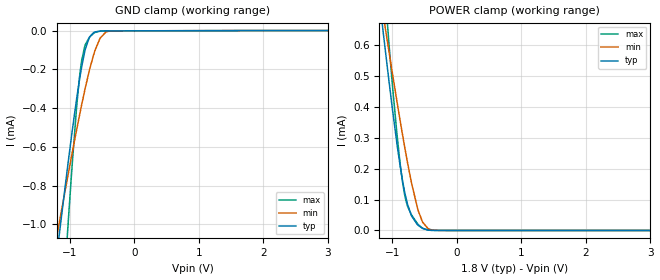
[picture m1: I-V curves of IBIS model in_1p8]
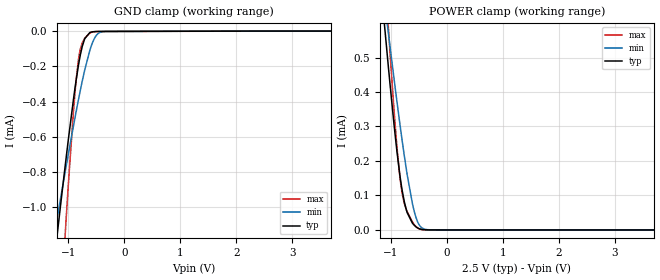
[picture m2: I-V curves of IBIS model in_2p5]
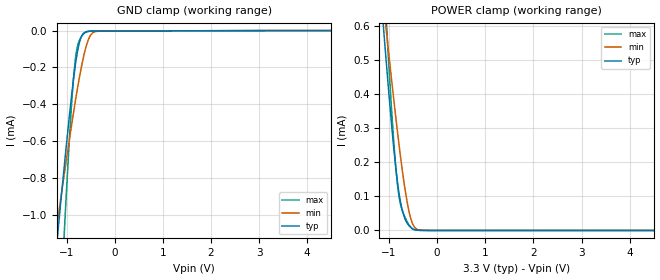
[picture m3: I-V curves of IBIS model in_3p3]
| Texas Instruments Incorporated
| High Speed, Robust EMC Reinforced Dual-Channel Digital Isolators
[IBIS Ver]   4.1
[File name]   iso6521.ibs
[File Rev]   1.0
[Date]   11/6/2023
[Source]
| Texas Instruments Incorporated.
| Analog-eLab Design Center, HPA
| 12500 TI Blvd
| Dallas, TX -75243
[Notes]   Revision History:
| Rev 1.0: 11/6/2023
| - Initial version of the model
|* EXCEPTION:   *
|* - For in_* and en_* models there will be leakage current in   *
|*   GROUND clamp because of a resistor(RH2) connected to pad.   *
|* - For inf_* models there will be leakage current in POWER clamp  *
|*   because of a resistor(R1) connected to pad.   *
[Disclaimer]
| This model is designed as an aid for customers of Texas Instruments.
| TI and its licensors and suppliers make no warranties, either expressed
| or implied, with respect to this  model, including the warranties of
| merchantability or fitness for a particular purpose. The model is
| provided solely on an "as is" basis. The entire risk as to its quality
| and performance is with the customer.
[Copyright]
(C) Copyright 2016 Texas Instruments Incorporated.All rights reserved.
| Marketing part#   Digital Voltage Range   Package-type   #pins
| IS07721DW   2.25V-5.5V   SOIC   16
| IS07721DWR   2.25V-5.5V   SOIC   16
|  Component ISO6521 8-Pin REU DFN package
|  Part # ISO6521
[Component]   IS06521DFN
[Manufacturer]   TI
[Package]   |8 REU - DFN package
|   typ   min   max
R_pkg   0.0519   0.0296   0.0664
L_pkg   1.5958n   1.4642n   1.7808n
C_pkg   0.3172p   0.2996p   0.3431p
[Pin]  signal_name   model_name   R_pin   L_pin   C_pin
1   VCC1   POWER   0.03706  1.83239n  0.42768p
2   OUTA   OUT   0.07937  1.93924n  0.37453p
3   INB   IN   0.08295  1.99423n  0.37759p
4   GND1   GND   0.06024  2.20170n  0.40515p
5   GND2   GND   0.06024  2.22600n  0.40576p
6   OUTB   OUT   0.08295  1.99420n  0.37782p
7   INA   IN   0.07937  1.93924n  0.37472p
8   VCC2   POWER   0.03703  1.83026n  0.42888p
|  Component ISO6521F 8-Pin REU DFN package
|  Part # ISO6521F
[Component]   IS06521FDFN
[Manufacturer]   TI
[Package]   |8 REU - DFN package
|   typ   min   max
R_pkg   0.0519   0.0296   0.0664
L_pkg   1.5958n   1.4642n   1.7808n
C_pkg   0.3172p   0.2996p   0.3431p
[Pin]  signal_name   model_name   R_pin   L_pin   C_pin
1   VCC1   POWER   0.03706  1.83239n  0.42768p
2   OUTA   OUT   0.07937  1.93924n  0.37453p
3   INB   INF   0.08295  1.99423n  0.37759p
4   GND1   GND   0.06024  2.20170n  0.40515p
5   GND2   GND   0.06024  2.22600n  0.40576p
6   OUTB   OUT   0.08295  1.99420n  0.37782p
7   INA   INF   0.07937  1.93924n  0.37472p
8   VCC2   POWER   0.03703  1.83026n  0.42888p
|   Model Selectors
[Model Selector] IN
in_1p8   1.8V digital Input
in_2p5   2.5V digital Input
in_3p3   3.3V digital Input
in_5   5.0V digital Input
[Model Selector] INF
inf_1p8   1.8V digital Input
inf_2p5   2.5V digital Input
inf_3p3   3.3V digital Input
inf_5   5.0V digital Input
[Model Selector] OUT
out_1p8   1.8V digital Output
out_2p5   2.5V digital Output
out_3p3   3.3V digital Output
out_5   5.0V digital Output
| Models and submodels in the file (12): in_1p8 (Input), in_2p5 (Input), in_3p3 (Input), in_5 (Input), inf_1p8 (Input), inf_2p5 (Input), inf_3p3 (Input), inf_5 (Input), out_1p8 (3-state), out_2p5 (3-state), out_3p3 (3-state), out_5 (3-state)
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|   in_2p5 Model
[Model]   in_1p8
Model_type   Input
Vinl = 0.54
Vinh = 1.26
|   typ   min   max
C_comp   0.00095pF   0.00076pF   0.0142pF
[Model spec]
|subparameter
Vinl   0.54   0.513   0.567
Vinh   1.26   1.197   1.323
| Where nom  PVT is Nominal Process, 2.5V, 27C
|   Fast PVT is Strong Process,  2.75V, -55C
|   Slow PVT is Weak Process,   2.25V, 150C
[Voltage Range]   1.8   1.71   1.89
|Ambient Temperature   25   125   -55
|Junction Temperature
[Temperature Range]   27   150   -40
[Power Clamp Reference]   1.8   1.71   1.89
[GND Clamp Reference]   0   0   0
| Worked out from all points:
|   GND clamp passes 1 mA (typ) near -1.14 V on its own axis
|   POWER clamp passes 1 mA (typ) near -1.34 V on its own axis
[GND Clamp]
|   Voltage   I(typ)   I(min)   I(max)
-1.8V     -2.874mA   -2.195mA   -5.336mA
-1.184V   -1.11mA    -1.03mA    -1.821mA
-1.163V   -1.051mA   -990.6uA   -1.705mA
-1.028V   -686uA     -745.6uA   -1.004mA
-898.2mV  -361.3uA   -518.9uA   -411.1uA
-828mV    -209.5uA   -402uA     -181.4uA
-757.8mV  -93.79uA   -292.1uA   -71.12uA
-698.4mV  -36.2uA    -207.5uA   -35.59uA
-633.6mV  -10.97uA   -127.9uA   -14.52uA
-531mV    -2.469uA   -39.62uA   -2.975uA
-369mV    -1.445uA   -2.669uA   -1.543uA
3.6V      0A         0A         0A
[POWER Clamp]
|   Voltage   I(typ)   I(min)   I(max)
-1.8V     1.872mA    1.618mA    2.869mA
-1.179V   709.8uA    751.5uA    957.6uA
-1.055V   490uA      584.3uA    612.9uA
-919.8mV  269uA      408.1uA    296.9uA
-871.2mV  199.5uA    346.9uA    204.2uA
-817.2mV  133.9uA    281.2uA    125.6uA
-768.6mV  88.65uA    224.9uA    81.75uA
-703.8mV  48uA       155.6uA    51.14uA
-612mV    19.26uA    74.45uA    22.69uA
-531mV    6.785uA    27.03uA    7.136uA
-293.4mV  209.8nA    425.9nA    202.8nA
3.6V      0A         0A         0A
|   in_2p5 Model
[Model]   in_2p5
Model_type   Input
Vinl = 0.75
Vinh = 1.75
|   typ   min   max
C_comp   0.00095pF   0.00076pF   0.015pF
|  Where Nom  PVT is Nominal Process, 2.5V,   27C
|   Fast PVT is Strong Process,  2.25,   -340C
|   Slow PVT is Weak Process,   2.75V,  150C
[Model spec]
|subparameter
Vinl   0.75   0.675   0.825
Vinh   1.75   1.575   1.925
[Voltage Range]   2.5   2.25   2.75
|Junction Temperature
[Temperature Range]   27   150   -40
[Power Clamp Reference]   2.5   2.25   2.75
[GND Clamp Reference]   0   0   0
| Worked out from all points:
|   GND clamp passes 1 mA (typ) near -1.14 V on its own axis
[GND Clamp]
|   Voltage   I(typ)   I(min)   I(max)
-2.5V     -4.931mA   -3.55mA    -9.461mA
-1.232V   -1.244mA   -1.119mA   -2.084mA
-1.12V    -933.5uA   -912.3uA   -1.477mA
-1.038V   -711.7uA   -763uA     -1.052mA
-910mV    -389.1uA   -539.1uA   -459uA
-820mV    -194.3uA   -389.1uA   -163uA
-782.5mV  -129.3uA   -329.8uA   -97.62uA
-707.5mV  -42.82uA   -219.9uA   -40.05uA
-617.5mV  -8.649uA   -110.7uA   -11.7uA
-497.5mV  -2.387uA   -23.45uA   -2.737uA
-355mV    -1.896uA   -2.716uA   -2.116uA
5V        0A         0A         0A
[POWER Clamp]
|   Voltage   I(typ)   I(min)   I(max)
-2.5V     3.216mA    2.616mA    5.089mA
-1.113V   590.9uA    661.5uA    768.3uA
-1.067V   512uA      601.2uA    646.2uA
-1.03V    447.5uA    551.4uA    549.6uA
-902.5mV  243.4uA    386.1uA    262.1uA
-842.5mV  162.8uA    311.7uA    158.7uA
-805mV    121.3uA    266.8uA    112.2uA
-722.5mV  57.6uA     174.8uA    58.38uA
-617.5mV  20.43uA    78.61uA    24.1uA
-497.5mV  3.903uA    15.71uA    3.749uA
-257.5mV  171.2nA    276.9nA    172.3nA
5V        0A         0A         0A
|   in_3p3 Model
[Model]   in_3p3
Model_type   Input
Vinl = 0.99
Vinh = 2.31
|   typ   min   max
C_comp   0.00096pF   0.00076pF   0.016pF
|  Where Nom  PVT is Nominal Process, 3.3V,   27C
|   Fast PVT is Strong Process,  3.6,   -40C
|   Slow PVT is Weak Process,   3.0V,   150C
[Model spec]
|subparameter
Vinl   0.99   0.9   1.08
Vinh   2.31   2.1   2.52
[Voltage Range]   3.3   3   3.6
|Junction Temperature
[Temperature Range]   27   150   -40
[Power Clamp Reference]   3.3   3   3.6
[GND Clamp Reference]   0   0   0
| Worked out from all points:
|   GND clamp passes 1 mA (typ) near -1.14 V on its own axis
|   POWER clamp passes 1 mA (typ) near -1.34 V on its own axis
[GND Clamp]
|   Voltage   I(typ)   I(min)   I(max)
-3.3V     -7.303mA   -5.115mA   -14.21mA
-1.211V   -1.185mA   -1.08mA    -1.967mA
-1.152V   -1.02mA    -970.3uA   -1.646mA
-1.112V   -912uA     -897.9uA   -1.436mA
-1.033V   -699.6uA   -754.9uA   -1.03mA
-904.2mV  -375.5uA   -529.2uA   -435.5uA
-815.1mV  -185.3uA   -381.3uA   -152.7uA
-716.1mV  -49.91uA   -231.9uA   -44.58uA
-597.3mV  -6.774uA   -90.92uA   -9.051uA
-458.7mV  -2.634uA   -12.21uA   -2.924uA
-260.7mV  -2.357uA   -2.487uA   -2.627uA
6.6V      0A         0A         0A
[POWER Clamp]
|   Voltage   I(typ)   I(min)   I(max)
-3.3V     4.765mA    3.768mA    7.646mA
-1.132V   625.4uA    687.7uA    822.6uA
-1.102V   572.7uA    647.7uA    739.9uA
-1.082V   538uA      621.1uA    686uA
-1.023V   435.6uA    542.1uA    532.2uA
-894.3mV  231.5uA    375.8uA    246.2uA
-805.2mV  121.5uA    267uA      112.4uA
-716.1mV  54.13uA    168.1uA    55.82uA
-617.1mV  20.34uA    78.3uA     23.99uA
-547.8mV  8.703uA    34.54uA    9.499uA
-468.6mV  2.306uA    9.387uA    2.038uA
6.6V      0A         0A         0A
